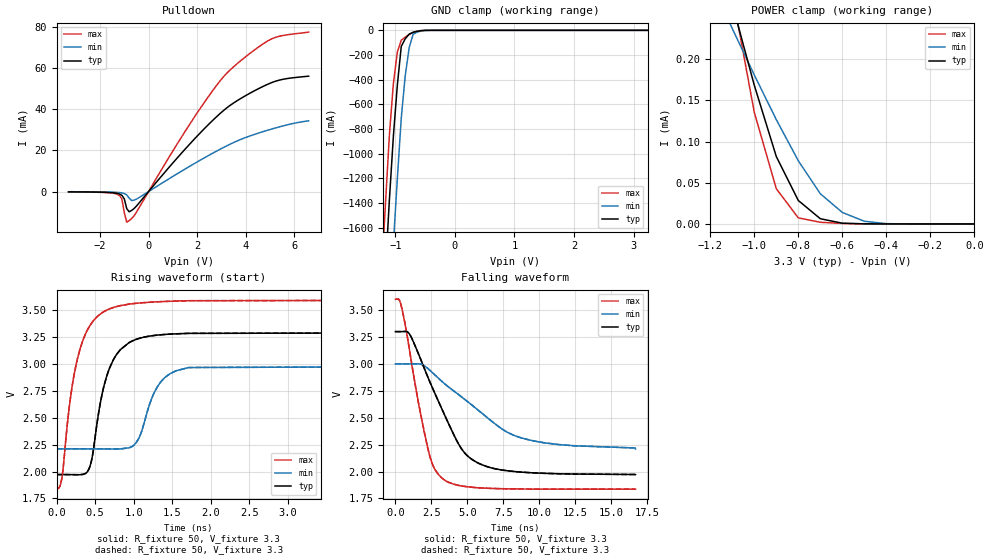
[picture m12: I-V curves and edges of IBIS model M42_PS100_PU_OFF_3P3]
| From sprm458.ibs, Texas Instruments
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|   Model Cell M42_PS100_PU_OFF_3P3
|IDG09_OUM42_PS100_PU_OFF_3P3
[Model]   M42_PS100_PU_OFF_3P3
Model_type   I/O_open_drain
Polarity   Non-Inverting
Enable   Active-Low
Vinl =  0.8V
Vinh =  2V
Cref =  15pF
Rref =  100.00M
Vref =  0V
Vmeas =  1.65
C_comp   4.770p   4.586p   5.631p
[Model Spec]
Vinl   0.8V   0.8V   0.8V
Vinh   2V   2V   2V
[Temperature Range]   25   125   -40
[Voltage Range]   3.3   3   3.6
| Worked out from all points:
|   slope of the pulldown table from 0 to 0.495 V, typ, clamps not added: 71.1 ohm
|   GND clamp passes 1 mA (typ) near -0.52 V on its own axis
|   POWER clamp passes 1 mA (typ) near -1.78 V on its own axis
|   rising waveform, R_fixture 50, V_fixture 3.3: 20-80 % time 250ps typ, 264ps min, 252ps max; typ from 1.97 V to 3.3 V
|   rising waveform, R_fixture 50, V_fixture 3.3: 20-80 % time 250ps typ, 264ps min, 252ps max; typ from 1.97 V to 3.3 V
|   falling waveform, R_fixture 50, V_fixture 3.3: 20-80 % time 2.69ns typ, 4.54ns min, 1.47ns max; typ from 3.3 V to 1.97 V
|   falling waveform, R_fixture 50, V_fixture 3.3: 20-80 % time 2.69ns typ, 4.54ns min, 1.47ns max; typ from 3.3 V to 1.97 V
| Nom Voltages:
|   VDD=1.1, VDDS=3.3, VSS=0, VSSS=0
| Min Voltages:
|   VDD=1, VDDS=3, VSS=0, VSSS=0
| Max Voltages:
|   VDD=1.2, VDDS=3.6, VSS=0, VSSS=0
[POWER_clamp]
|   voltage   I(typ)   I(min)   I(max)
-3.3V     2.695mA    1.572mA    4.067mA
-1.1V     266.9uA    237.2uA    279.9uA
-1.067V   234.1uA    218.4uA    231.7uA
-1V       168.4uA    180.8uA    135.5uA
-900mV    81.82uA    126.6uA    42.76uA
-800mV    28.47uA    76.69uA    7.358uA
-700mV    6.356uA    36.67uA    2.023uA
-600mV    885nA      13.95uA    630.3nA
-500mV    144.6nA    3.261uA    75.42nA
-400mV    11.31nA    356.8nA    2.764nA
0V        95.94pA    13.84nA    1.15pA
[Pulldown]
|   voltage   I(typ)   I(min)   I(max)
-3.3V     -125.5uA   -69.78uA   -154uA
-1.3V     -854.4uA   -377.5uA   -1.265mA
-1.1V     -1.818mA   -637.4uA   -3.603mA
-1V       -3.544mA   -939uA     -10.26mA
-900mV    -8.266mA   -1.615mA   -14.87mA
-800mV    -9.812mA   -3.181mA   -14.12mA
-700mV    -9.167mA   -4.347mA   -13.12mA
-500mV    -7.047mA   -3.656mA   -10mA
1.7V      23.11mA    12.3mA     32.76mA
3.2V      40.42mA    22.07mA    57.19mA
5V        52.57mA    30.11mA    73.74mA
6.6V      56.07mA    34.37mA    77.47mA
[GND_clamp]
|   voltage   I(typ)   I(min)   I(max)
-3.3V     -22.64A    -23.49A    -22.17A
-1.233V   -2.55A     -3.487A    -2.002A
-1.167V   -1.958A    -2.887A    -1.417A
-1.1V     -1.378A    -2.296A    -853.3mA
-1.033V   -864.2mA   -1.736A    -435.2mA
-966.7mV  -447.9mA   -1.207A    -177.1mA
-900mV    -129.5mA   -710.5mA   -79.22mA
-833.3mV  -68.39mA   -365.8mA   -54.87mA
-766.7mV  -30.48mA   -139.2mA   -33.79mA
-700mV    -15.74mA   -30.55mA   -15.98mA
-500mV    -441.4uA   -1.393mA   -154.5uA
3.233V    93.53pA    23.72nA    954.8fA
[Ramp]
| variable   typ   min   max
dV/dt_f 0.79816213/2.6888806n 0.47459191/4.5449174n  1.0598264/1.4680225n
dV/dt_r 15.722938m/0.10150889n 12.195979m/0.16710668n 17.258143m/68.630381p
R_load = 50
[Rising Waveform]
R_fixture = 50
V_fixture = 3.3
V_fixture_min = 3
V_fixture_max = 3.6
|   time   V(typ)   V(min)   V(max)
0s        1.971V     2.21V      1.836V
68.43ps   1.972V     2.21V      1.934V
205.9ps   1.971V     2.21V      2.807V
350ps     1.975V     2.21V      3.232V
451.9ps   2.097V     2.21V      3.374V
672.3ps   2.931V     2.209V     3.505V
940.5ps   3.196V     2.22V      3.553V
1.349ns   3.268V     2.829V     3.576V
1.711ns   3.282V     2.965V     3.585V
16.67ns   3.3V       3V         3.6V
[Rising Waveform]
R_fixture = 50
V_fixture = 3.3
V_fixture_min = 3
V_fixture_max = 3.6
|   time   V(typ)   V(min)   V(max)
0s        1.971V     2.21V      1.836V
68.43ps   1.972V     2.21V      1.934V
205.9ps   1.971V     2.21V      2.807V
350ps     1.975V     2.21V      3.232V
451.9ps   2.097V     2.21V      3.374V
672.3ps   2.931V     2.209V     3.505V
940.5ps   3.196V     2.22V      3.553V
1.349ns   3.268V     2.829V     3.576V
1.711ns   3.282V     2.965V     3.585V
16.67ns   3.3V       3V         3.6V
[Falling Waveform]
R_fixture = 50
V_fixture = 3.3
V_fixture_min = 3
V_fixture_max = 3.6
|   time   V(typ)   V(min)   V(max)
0s        3.3V       3V         3.6V
271.4ps   3.3V       3V         3.593V
493.5ps   3.3V       3V         3.488V
1.031ns   3.266V     3V         3.085V
2.33ns    2.853V     2.948V     2.173V
3.271ns   2.568V     2.832V     1.935V
4.744ns   2.183V     2.677V     1.863V
6.411ns   2.043V     2.497V     1.844V
9.281ns   1.99V      2.294V     1.837V
16.67ns   1.971V     2.21V      1.836V
[Falling Waveform]
R_fixture = 50
V_fixture = 3.3
V_fixture_min = 3
V_fixture_max = 3.6
|   time   V(typ)   V(min)   V(max)
0s        3.3V       3V         3.6V
271.4ps   3.3V       3V         3.593V
493.5ps   3.3V       3V         3.488V
1.031ns   3.266V     3V         3.085V
2.33ns    2.853V     2.948V     2.173V
3.271ns   2.568V     2.832V     1.935V
4.744ns   2.183V     2.677V     1.863V
6.411ns   2.043V     2.497V     1.844V
9.281ns   1.99V      2.294V     1.837V
16.67ns   1.971V     2.21V      1.836V
